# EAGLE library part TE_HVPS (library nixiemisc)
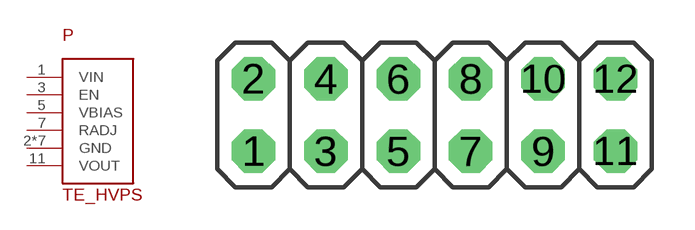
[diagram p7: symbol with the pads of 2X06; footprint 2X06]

Designator prefix P

## TE_HVPSVERTICAL  [2X06]
1  VIN  pwr
2  GND  pwr
3  EN  pas
4  GND  pwr
5  VBIAS  pwr
6  GND  pwr
7  RADJ  pas
8  GND  pwr
9  GND  pwr
10  GND  pwr
11  VOUT  pwr
12  GND  pwr

## Footprint 2X06 (pad centres in mm)
PIN HEADER
drill 1.016 octagon: 1 -6.35,-1.27; 2 -6.35,1.27; 3 -3.81,-1.27; 4 -3.81,1.27; 5 -1.27,-1.27; 6 -1.27,1.27; 7 1.27,-1.27; 8 1.27,1.27; 9 3.81,-1.27; 10 3.81,1.27; 11 6.35,-1.27; 12 6.35,1.27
